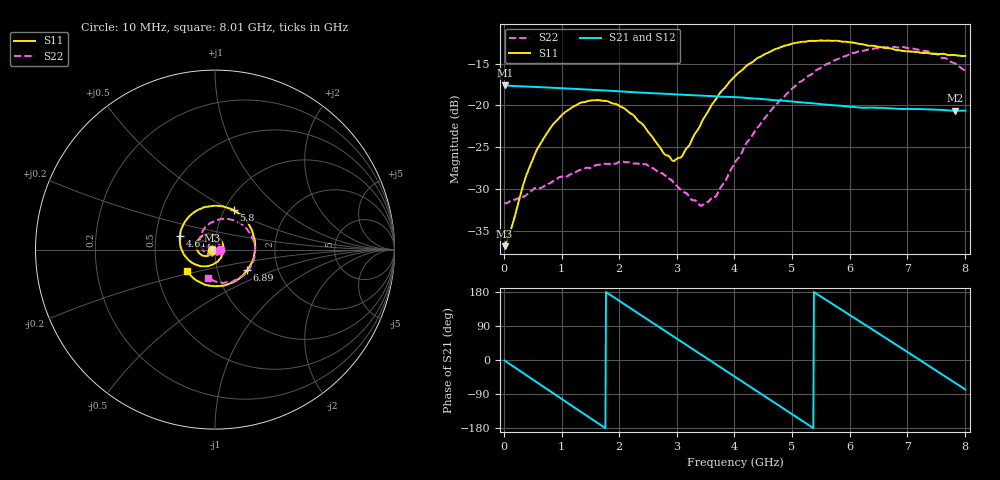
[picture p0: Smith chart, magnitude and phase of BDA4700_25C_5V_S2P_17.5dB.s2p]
!Agilent Technologies,E5071B,MY42404982,A.09.10
!Date: Mon Oct 20 13:35:03 2025
!Data & Calibration Information:
!Freq	S11:SOLT2(ON)	S21:SOLT2(ON)	S12:SOLT2(ON)	S22:SOLT2(ON)
# Hz S RI R 50
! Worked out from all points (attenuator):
!   801 points, 10 MHz to 8.01 GHz, reference 50 ohm
!   highest |S21| = -17.60 dB at 20 MHz (marker M1); lowest = -20.6 dB at 7.83 GHz (marker M2)
!   lowest |S11| = -36.8 dB at 10 MHz (marker M3), VSWR 1.03, Z = 48.6 - j0.142 ohm
!   |S11| at or under -10 dB: start of sweep to end of sweep
!   |S22| runs from -32.0 to -13.0 dB; largest |S21 - S12| = 0.00094
!   S11 on the Smith chart (normalised r, x): 10 MHz: 0.97, -0.00; 4.61 GHz: 0.67, +0.10; 5.8 GHz: 1.10, +0.52; 6.89 GHz: 1.39, -0.34; 8.01 GHz: 0.71, -0.18
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1e7  -0.0143 -0.00146  0.1318 -0.00291  0.1318 -0.00302  0.026 -0.00091
2e7  -0.0147 -0.00221  0.1317 -0.00507  0.1317 -0.00548  0.0259 -0.0011
3.7e8  -0.0254 -0.0263  0.1017 -0.0807  0.1016 -0.0808  0.0215 -0.0191
5.9e8  -0.0428 -0.036  0.0625 -0.1126  0.0624 -0.1127  0.0133 -0.0292
9.9e8  -0.0829 -0.0246  -0.0258 -0.1242  -0.0259 -0.1242  -0.015 -0.0342
1.35e9  -0.1032 0.0142  -0.0933 -0.0831  -0.0934 -0.0833  -0.0376 -0.017
2.07e9  -0.0414 0.0874  -0.1039 0.0621  -0.104 0.0622  -0.0287 0.036
2.68e9  0.0395 0.042  0.00366 0.1179  0.00365 0.1178  0.0168 0.0362
2.92e9  0.0469 0.00145  0.0505 0.1051  0.0505 0.105  0.0275 0.0223
3.05e9  0.0433 -0.0222  0.0724 0.0906  0.072 0.091  0.0293 0.0118
3.43e9  -0.00488 -0.0791  0.1113 0.0272  0.1113 0.0272  0.0181 -0.0174
3.69e9  -0.0592 -0.0932  0.1107 -0.0237  0.1108 -0.0241  -0.00227 -0.0288
4.01e9  -0.1314 -0.0704  0.0804 -0.078  0.0805 -0.0778  -0.0363 -0.0272
4.61e9  -0.1951 0.074  -0.0265 -0.1049  -0.0264 -0.105  -0.082 0.0395
5.35e9  -0.0477 0.2384  -0.1029 -0.00412  -0.103 -0.00439  -0.0135 0.1537
5.8e9  0.1036 0.2201  -0.0742 0.0665  -0.0742 0.0667  0.0905 0.1668
6.23e9  0.2049 0.109  -0.0112 0.0962  -0.0103 0.0964  0.1835 0.1067
6.68e9  0.2142 -0.0494  0.0583 0.0764  0.0585 0.0764  0.2218 -0.00848
6.89e9  0.1793 -0.1153  0.0805 0.0508  0.0808 0.0506  0.2125 -0.0679
7.35e9  0.0436 -0.2016  0.0924 -0.021  0.0924 -0.0212  0.1326 -0.1643
7.83e9  -0.1141 -0.1647  0.0465 -0.0804  0.0464 -0.0806  0.00436 -0.1781
8.01e9  -0.1561 -0.1216  0.0194 -0.0909  0.0195 -0.0909  -0.0377 -0.1558
